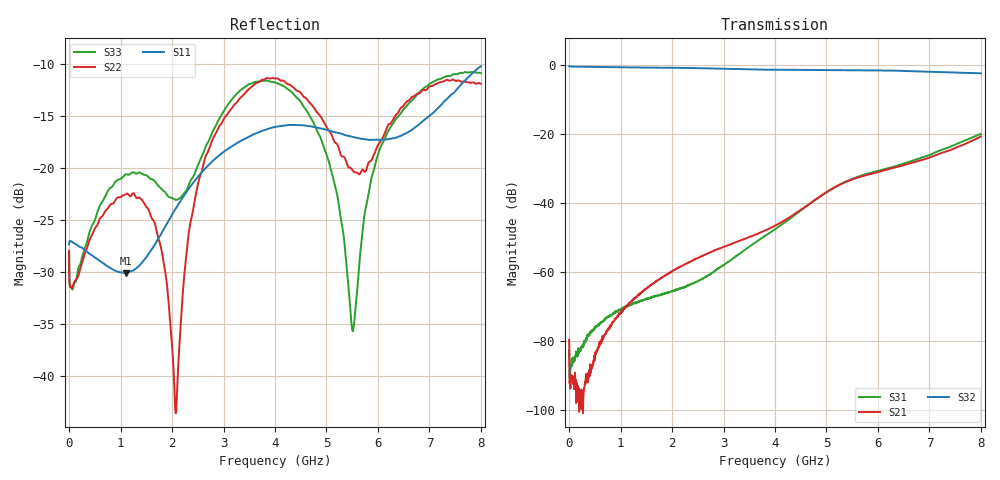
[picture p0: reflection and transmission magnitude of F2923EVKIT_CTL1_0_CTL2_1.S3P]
! Integrated Device Technology
! Corporate Headquarters
! 6024 Silver Creek Valley Road
! San Jose, CA 95138  USA
! Phone:  1-408-284-8200
! Toll Free:  1-800-223-1366
! Webpage:  http://www.idt.com/
! Timing and RF Division
! 515 Groton Road, Suite 102
! Westford, MA 01886-6024
! Device:  F2923
! Description: Constant Impedance Kz SP2T RF Switch
! Frequency:  0.3 MHz to 8 GHz
! Package:  4 mm x 4 mm QFN Plastic Package: 20 pin
! Ports:  3 RF, 3 DC
!  Pin  1  = GND
!  Pin  2  = GND
!  Pin  3  = RF1  = Port 1
!  Pin  4  = GND
!  Pin  5  = GND
!  Pin  6  = GND
!  Pin  7  = GND
!  Pin  8  = RF_COM  = Port 3
!  Pin  9  = GND
!  Pin  10  = GND
!  Pin  11  = GND
!  Pin  12  = GND
!  Pin  13  = RF2  = Port 2
!  Pin  14  = GND
!  Pin  15  = NC
!  Pin  16  = CTL2
!  Pin  17  = CTL1
!  Pin  18  = NC
!  Pin  19  = ModeCTL
!  Pin  20  = VCC
!  EP  = GND
! State:  RF2 On
! Voltage:  VCC  = +3.3 V
!  CTL1  = 0 V (Logic LOW)
!  CTL2  = 3.3 V (Logic HIGH)
! Data:  The device was measured on the F2923 EVKit
!  using a calibrated network analyzer.
!  The results below include the EVKit RF connector and
!		PCB loss effects. The reference plane is at
!  the SMA coaxial interface. Refer to the separate
!  measured thru line.s2p file for connector and PCB loss
!  and effects.
! Misc:
! Date Measured:  2017-8-14
! Date:  2017-8-14  SPJ
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# Hz S dB R 50
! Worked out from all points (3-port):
!   1601 points, 300 kHz to 8 GHz, reference 50 ohm
!   strongest paths, dB at 300 kHz, 2 GHz, 4 GHz, 6 GHz, 8 GHz:
!     S32: -0.3, -0.8, -1.4, -1.5, -2.4
!     S21: -79.6, -59.7, -46.6, -31.0, -20.7
!     S31: -82.6, -65.4, -47.6, -30.7, -19.9
!   lowest |S11| = -30.1 dB at 1.11 GHz (marker M1), VSWR 1.06, Z = 47.3 + j1.33 ohm
!   |S11| at or under -10 dB: start of sweep to end of sweep
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300000  -27.37 179.3  -95.85 -107.7  -74.59 -109.2
        -79.63 122.8  -27.97 -10.1  -0.32 0.1
        -82.59 -131.0  -0.33 0.1  -28.08 -8.9
1.110258e9  -30.11 153.2  -70.09 56.3  -69.92 3.4
            -69.91 54.9  -22.51 160.3  -0.68 -120.0
            -69.91 1.8  -0.67 -120.0  -20.62 -177.9
2.075222e9  -23.90 148.4  -59.13 -27.7  -65.32 -50.6
            -59.14 -27.5  -43.55 -40.0  -0.80 136.6
            -64.96 -50.2  -0.80 136.6  -23.09 134.6
2.500206e9  -20.88 129.3  -55.92 -65.4  -62.75 -65.8
            -55.93 -65.8  -21.65 -170.4  -0.89 90.7
            -62.62 -66.0  -0.89 90.8  -19.80 136.0
4.00015e9  -16.07 46.1  -46.57 171.1  -47.64 -162.1
           -46.57 171.0  -11.41 26.2  -1.36 -69.0
           -47.58 -161.7  -1.37 -69.0  -11.79 14.1
4.965114e9  -16.30 -10.0  -37.19 81.3  -37.15 102.1
            -37.17 81.3  -15.72 -54.2  -1.45 -172.3
            -37.24 102.0  -1.42 -172.4  -18.23 -82.4
5.510093e9  -17.03 -38.0  -33.02 13.4  -33.08 33.4
            -33.11 13.8  -20.26 -73.8  -1.49 129.0
            -32.96 32.8  -1.51 128.8  -35.71 -55.4
5.835081e9  -17.32 -53.7  -31.59 -26.0  -31.44 -7.2
            -31.67 -26.4  -19.41 -76.2  -1.54 93.7
            -31.32 -6.1  -1.52 93.3  -22.04 3.7
6.760046e9  -15.99 -101.0  -27.94 -129.1  -27.28 -108.6
            -27.92 -128.8  -12.89 -127.4  -1.82 -8.1
            -27.29 -109.4  -1.84 -8.1  -12.97 -90.7
8e9  -10.23 152.0  -20.78 95.5  -19.81 112.5
     -20.66 94.1  -11.92 95.6  -2.42 -145.2
     -19.95 113.4  -2.40 -145.5  -10.90 132.2
